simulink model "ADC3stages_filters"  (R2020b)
settings: Solver=VariableStepAuto  StartTime=0.0  StopTime=100e-3  RelTol=1e-3
libraries: ee_lib x8, fl_lib x5, nesl_utility x4, simulink_extras x2, dspmlti4 x2, simulink x1

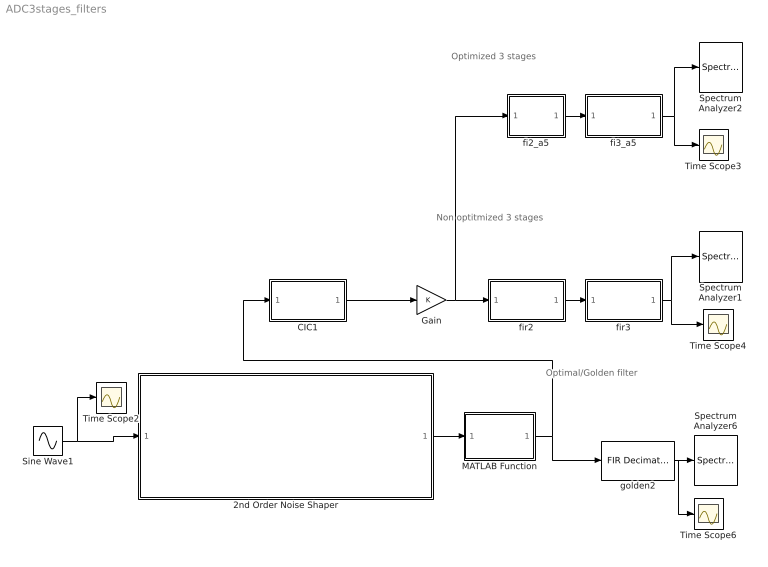
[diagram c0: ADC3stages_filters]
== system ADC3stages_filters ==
  note: Optimized 3 stages
  note: Non optitmized 3 stages
  note: Optimal/Golden filter
  2nd Order Noise Shaper : Subsystem
  CIC1 : Subsystem  Tag=BlockMethodSubSystem
  Gain : Gain  ParamDataTypeStr=int16
  MATLAB Function : MATLAB Function  TreatAsAtomicUnit=on
  Sine Wave1 : Sin  Amplitude=0.5  Bias=0.5  Frequency=2*pi*2000  SampleTime=0
  Spectrum Analyzer1 : SpectrumAnalyzer
  Spectrum Analyzer2 : SpectrumAnalyzer
  Spectrum Analyzer6 : SpectrumAnalyzer  Commented=on
  Time Scope{2..4,6} (4 alike) : Scope
  fi2_a5 : Subsystem  Tag=FilterWizardSubSystem
  fi3_a5 : Subsystem  Tag=FilterWizardSubSystem
  fir2 : Subsystem  Tag=FilterWizardSubSystem
  fir3 : Subsystem  Tag=FilterWizardSubSystem
  golden2 : dspmlti4/FIR Decimation  Tag=BlockMethodSubSystem  FilterSource=Dialog parameters  h=[-9.28934945917742932e-09 -2.06150874537475163e-09 -2.28946243433772473e-09 -2.53402570041462021e-09 -2.79572593785659298e-09 -3.07556170283654811e-09 -3.37426400279055493e-09 -3.69267761653814601e-09 -4.0317656513874688e-09 -4.39228892641005716e-09 -4.77551823656375575e-09 -5.18221175819345824e-09 -5.6139960130665323e-09 -6.07162645637982626e-09 -6.55700619397832109e-09 -7.07075410921223467e-09 -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  D=128  filtStruct=Direct form  FilterObject=FDECIM  InputProcessing=Columns as channels (frame based)  framing=Allow multirate processing  inputOffset=0  outputBufInitCond=0  roundingMode=Floor  overflowMode=off  firstCoeffDataTypeStr=Inherit: Same word length as input  firstCoeffMin=[]  firstCoeffMax=[]  firstCoeffLastDataTypeStr=Inherit: Same word length as input  outputDataTypeStr=Inherit: Same as accumulator  outputMin=[]  outputMax=[]  outputLastDataTypeStr=Inherit: Same as accumulator
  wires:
  Sine Wave1/1 -> 2nd Order Noise Shaper/1(input0), Time Scope2/1
  2nd Order Noise Shaper/1(u) -> MATLAB Function/1(u)
  golden2/1 -> Time Scope6/1, Spectrum Analyzer6/1
  MATLAB Function/1(y) -> CIC1/1(y), golden2/1
  fir2/1(Output) -> fir3/1(Input)
  fir3/1(Output) -> Spectrum Analyzer1/1, Time Scope4/1
  fi2_a5/1(Output) -> fi3_a5/1(Input)
  fi3_a5/1(Output) -> Spectrum Analyzer2/1, Time Scope3/1
  CIC1/1(Input) -> Gain/1
  Gain/1 -> fi2_a5/1(Input), fir2/1(Input)

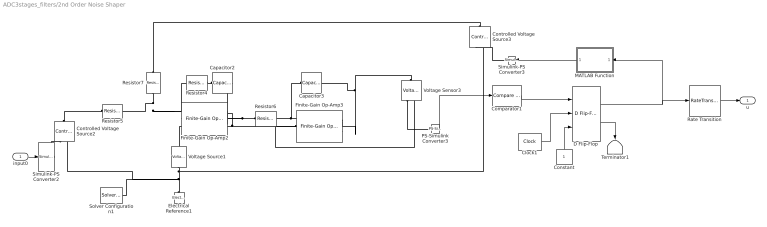
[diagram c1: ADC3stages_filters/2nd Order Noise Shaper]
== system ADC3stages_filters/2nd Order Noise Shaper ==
  input0 : Inport
  Capacitor2 : ee_lib/Passive/Capacitor  cap_option=0  c=100 pF  Cvec=[1e-05, 1e-06] F  Vvec=[0, 10] V  CV_table_symmetry=1  f_vec=[1, 10] kHz  DFext_vec=[.8, 1.2]  C_tol=5  enable_C_tol=0  tol_distribution=1  nSigma=4  r=1e-9 Ohm  g=0 1/Ohm  averaging_period=0 s  enable_operating_limits=0  operating_limit_action=2  max_working_voltage_range=[-25, 25] V  power_rating=1 W  enable_faults=0  fault_action=1  Cscale_faulted=100  R_faulted=1e-3 Ohm  G_faulted=0 1/Ohm  tau_fault=1e-3 s  enable_temporal_fault=0  t_fault=1 s  enable_behavioral_fault=0  max_permissible_voltage_range=[-100, 100] V  t_fail_on_voltage=1 s  i_specify=off  i_priority=None  i=0 A  i_nominal_specify=off  i_nominal_unit=A  i_nominal_value=1  v_specify=off  v_priority=None  v=0 V  v_nominal_specify=off  v_nominal_unit=V  v_nominal_value=1  vc_specify=off  vc_priority=High  vc=0 V  vc_nominal_specify=off  vc_nominal_unit=V  vc_nominal_value=1
  Capacitor3 : ee_lib/Passive/Capacitor  cap_option=0  c=100 pF  Cvec=[1e-05, 1e-06] F  Vvec=[0, 10] V  CV_table_symmetry=1  f_vec=[1, 10] kHz  DFext_vec=[.8, 1.2]  C_tol=5  enable_C_tol=0  tol_distribution=1  nSigma=4  r=1e-6 Ohm  g=0 1/Ohm  averaging_period=0 s  enable_operating_limits=0  operating_limit_action=2  max_working_voltage_range=[-25, 25] V  power_rating=1 W  enable_faults=0  fault_action=1  Cscale_faulted=100  R_faulted=1e-3 Ohm  G_faulted=0 1/Ohm  tau_fault=1e-3 s  enable_temporal_fault=0  t_fault=1 s  enable_behavioral_fault=0  max_permissible_voltage_range=[-100, 100] V  t_fail_on_voltage=1 s  i_specify=off  i_priority=None  i=0 A  i_nominal_specify=off  i_nominal_unit=A  i_nominal_value=1  v_specify=off  v_priority=None  v=0 V  v_nominal_specify=off  v_nominal_unit=V  v_nominal_value=1  vc_specify=off  vc_priority=High  vc=0 V  vc_nominal_specify=off  vc_nominal_unit=V  vc_nominal_value=1
  Clock1 : simulink_extras/Flip Flops/Clock  period=1/(6.25*1e6)
  Comparator1 : simulink/Logic and Bit Operations/Compare To Zero  relop=>=  OutDataTypeStr=boolean  ZeroCross=off
  Constant : Constant  SampleTime=0
  Controlled Voltage Source2 : fl_lib/Electrical/Electrical Sources/Controlled Voltage Source
  Controlled Voltage Source3 : fl_lib/Electrical/Electrical Sources/Controlled Voltage Source
  D Flip-Flop : simulink_extras/Flip Flops/D Flip-Flop
  Electrical Reference1 : fl_lib/Electrical/Electrical Elements/Electrical Reference
  Finite-Gain Op-Amp2 : ee_lib/Integrated Circuits/Finite-Gain Op-Amp  A=1000  Rin=1e6 Ohm  Rout=1 Ohm  Vmin=-1 V  Vmax=1 V  noise_mode=0  v_noise=30e-9 V/Hz^0.50000  noise_prm=1  i_noise=0.5e-12 A/Hz^0.50000  ip_noise=0.5e-12 A/Hz^0.50000  in_noise=0.5e-12 A/Hz^0.50000  sample_time=1e-3 s  repeatability=1  auto_seed_v=3499211588  auto_seed_ip=3890346746  auto_seed_in=545404223  user_seed_v=0  user_seed_ip=0  user_seed_in=0
  Finite-Gain Op-Amp3 : ee_lib/Integrated Circuits/Finite-Gain Op-Amp  A=1000  Rin=1e6 Ohm  Rout=1 Ohm  Vmin=-1 V  Vmax=1 V  noise_mode=0  v_noise=30e-9 V/Hz^0.50000  noise_prm=1  i_noise=0.5e-12 A/Hz^0.50000  ip_noise=0.5e-12 A/Hz^0.50000  in_noise=0.5e-12 A/Hz^0.50000  sample_time=1e-3 s  repeatability=1  auto_seed_v=3922919431  auto_seed_ip=2715962282  auto_seed_in=418932850  user_seed_v=0  user_seed_ip=0  user_seed_in=0
  MATLAB Function : MATLAB Function  TreatAsAtomicUnit=on
  PS-Simulink Converter3 : nesl_utility/PS-Simulink Converter  PhysicalDomain=network_engine_domain  SubClassName=ps_output  LeftPortType=input  RightPortType=output  PseudoPeriodic=off  Frequencies=[]  Unit=V  AffineConversion=off
  Rate Transition : RateTransition  OutPortSampleTime=1/(6.25e6)
  Resistor4 : fl_lib/Electrical/Electrical Elements/Resistor  R=4.304 kOhm  i_specify=off  i_priority=None  i=0 A  i_nominal_specify=off  i_nominal_unit=A  i_nominal_value=1  v_specify=off  v_priority=None  v=0 V  v_nominal_specify=off  v_nominal_unit=V  v_nominal_value=1
  Resistor5 : ee_lib/Passive/Resistor  R=4.304 kOhm  R_tol=5  enable_R_tol=0  tol_distribution=1  nSigma=4  enable_operating_limits=0  operating_limit_action=2  max_working_voltage=100 V  power_rating=1 W  enable_faults=0  fault_action=1  R_faulted=inf Ohm  enable_temporal_fault=0  t_fault=1 s  enable_behavioral_fault=0  max_permissible_current=1 A  t_fail_on_current=1 s  noise_mode=0  sample_time=1e-3 s  repeatability=1  auto_seed=1196140742  user_seed=0  Tdevice=25 degC  alpha=3.93e-3 1/K  Tmeas=25 degC  thermal_mass=100 J/K  power_derating_T1=70 degC  power_derating_T2=155 degC  operating_temperature_range_vec=[-50, 150] degC  temperature_specify=off  temperature_priority=High  temperature=298.15 K  temperature_nominal_specify=off  temperature_nominal_unit=K  temperature_nominal_value=1
  Resistor6 : ee_lib/Passive/Resistor  R=4.304 kOhm  R_tol=5  enable_R_tol=0  tol_distribution=1  nSigma=4  enable_operating_limits=0  operating_limit_action=2  max_working_voltage=100 V  power_rating=1 W  enable_faults=0  fault_action=1  R_faulted=inf Ohm  enable_temporal_fault=0  t_fault=1 s  enable_behavioral_fault=0  max_permissible_current=1 A  t_fail_on_current=1 s  noise_mode=0  sample_time=1e-3 s  repeatability=1  auto_seed=2348838240  user_seed=0  Tdevice=25 degC  alpha=3.93e-3 1/K  Tmeas=25 degC  thermal_mass=100 J/K  power_derating_T1=70 degC  power_derating_T2=155 degC  operating_temperature_range_vec=[-50, 150] degC  temperature_specify=off  temperature_priority=High  temperature=298.15 K  temperature_nominal_specify=off  temperature_nominal_unit=K  temperature_nominal_value=1
  Resistor7 : ee_lib/Passive/Resistor  R=4.304 kOhm  R_tol=5  enable_R_tol=0  tol_distribution=1  nSigma=4  enable_operating_limits=0  operating_limit_action=2  max_working_voltage=100 V  power_rating=1 W  enable_faults=0  fault_action=1  R_faulted=inf Ohm  enable_temporal_fault=0  t_fault=1 s  enable_behavioral_fault=0  max_permissible_current=1 A  t_fail_on_current=1 s  noise_mode=0  sample_time=1e-3 s  repeatability=1  auto_seed=4112460543  user_seed=0  Tdevice=25 degC  alpha=3.93e-3 1/K  Tmeas=25 degC  thermal_mass=100 J/K  power_derating_T1=70 degC  power_derating_T2=155 degC  operating_temperature_range_vec=[-50, 150] degC  temperature_specify=off  temperature_priority=High  temperature=298.15 K  temperature_nominal_specify=off  temperature_nominal_unit=K  temperature_nominal_value=1
  Simulink-PS Converter2 : nesl_utility/Simulink-PS Converter  PhysicalDomain=network_engine_domain  SubClassName=ps_input  LeftPortType=input  RightPortType=output  PseudoPeriodic=off  Frequencies=[]  NoiseDistribution=none  NoiseParameters=[]  Unit=1  AffineConversion=off  FilteringAndDerivatives=provide  SimscapeFilterOrder=1  InputFilterTimeConstant=0.001  UdotUserProvided=0
  Simulink-PS Converter3 : nesl_utility/Simulink-PS Converter  PhysicalDomain=network_engine_domain  SubClassName=ps_input  LeftPortType=input  RightPortType=output  PseudoPeriodic=off  Frequencies=[]  NoiseDistribution=none  NoiseParameters=[]  Unit=1  AffineConversion=off  FilteringAndDerivatives=provide  SimscapeFilterOrder=1  InputFilterTimeConstant=0.001  UdotUserProvided=0
  Solver Configuration1 : nesl_utility/Solver Configuration  PhysicalDomain=network_engine_domain  SubClassName=solver  LeftPortType=input  RightPortType=generic  Tones=[]  Harmonics=[]  SimulateNoise=off  Profile=off  UseLocalSampling=off  EnableSwitchedLinearOptims=on  FrequencyDomain=off  UseCCode=off  RelTol=0.001  AbsTol=1e-06  MinStep=1e-09  ToWorkspace=off  RevertToSquareIcSolve=off  NumHomotopyIterations=100  PhasorMode=off  PhasorModeNumHarmonics=1  DoDC=off  ResidualTolerance=1e-09  UseLocalSolver=off  LocalSolverChoice=NE_BACKWARD_EULER_ADVANCER  LocalSolverSampleTime=0.001  DoFixedCost=off  MaxNonlinIter=3  MaxModeIter=2  ComputeImpulses=off  ImpulseIterations=2  LinearAlgebra=auto  EquationFormulation=NE_TIME_EF  DelaysMemoryBudget=1024  AutomaticFiltering=on  FilteringTimeConstant=0.001  PartitionStorageMethod=AS_NEEDED  PartitionMemoryBudget=1024  PartitionMethod=ROBUST
  Terminator1 : Terminator
  Voltage Sensor3 : fl_lib/Electrical/Electrical Sensors/Voltage Sensor
  Voltage Source1 : ee_lib/Sources/Voltage Source  dc_voltage=0.5 V  ac_voltage=0 V  ac_shift=0 rad  ac_frequency=60 Hz  noise_mode=0  PSD=0 V^2/Hz  repeatability=1  auto_seed=4144164703  user_seed=0  sample_time=1e-3 s  i_specify=off  i_priority=None  i=0 A  i_nominal_specify=off  i_nominal_unit=A  i_nominal_value=1  v_specify=off  v_priority=None  v=0 V  v_nominal_specify=off  v_nominal_unit=V  v_nominal_value=1
  u : Outport
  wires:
  PS-Simulink Converter3/1 -> Comparator1/1
  Clock1/1 -> D Flip-Flop/2
  D Flip-Flop/1 -> MATLAB Function/1(u), Rate Transition/1
  Constant/1 -> D Flip-Flop/3
  MATLAB Function/1(y) -> Simulink-PS Converter3/1
  D Flip-Flop/2 -> Terminator1/1
  Comparator1/1 -> D Flip-Flop/1
  input0/1 -> Simulink-PS Converter2/1
  Rate Transition/1 -> u/1
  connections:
  Voltage Source1/RConn1 -- Controlled Voltage Source3/RConn2 -- Controlled Voltage Source2/RConn2 -- Solver Configuration1/RConn1 -- Electrical Reference1/LConn1
  Resistor6/LConn1 -- Capacitor2/RConn1 -- Finite-Gain Op-Amp2/RConn1
  Finite-Gain Op-Amp3/LConn1 -- Voltage Sensor3/RConn2 -- Voltage Source1/LConn1 -- Finite-Gain Op-Amp2/LConn1
  Simulink-PS Converter3/RConn1 -- Controlled Voltage Source3/RConn1
  Voltage Sensor3/LConn1 -- Capacitor3/RConn1 -- Finite-Gain Op-Amp3/RConn1
  Resistor7/RConn1 -- Resistor5/RConn1 -- Resistor4/LConn1 -- Finite-Gain Op-Amp2/LConn2
  Capacitor3/LConn1 -- Resistor6/RConn1 -- Finite-Gain Op-Amp3/LConn2
  Simulink-PS Converter2/RConn1 -- Controlled Voltage Source2/RConn1
  Voltage Sensor3/RConn1 -- PS-Simulink Converter3/LConn1
  Capacitor2/LConn1 -- Resistor4/RConn1
  Controlled Voltage Source2/LConn1 -- Resistor5/LConn1
  Controlled Voltage Source3/LConn1 -- Resistor7/LConn1

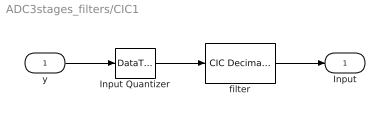
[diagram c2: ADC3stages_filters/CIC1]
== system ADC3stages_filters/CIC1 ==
  y : Inport
  Input Quantizer : DataTypeConversion  OutDataTypeStr=fixdt(1,16,15)  RndMeth=Round
  filter : dspmlti4/CIC Decimation  filtFrom=Dialog parameters  filtobj=CICDECIM  ftype=Decimator  R=32  M=1  N=2  filterInternals=Specify word lengths  BPS=[26 26 26 26]  FLPS=[15 15 15 15]  outputWordLength=14  outputFracLength=15  launchFVT=off  framing=Maintain input frame rate  RateOptions=Allow multirate processing
  Input : Outport
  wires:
  y/1 -> Input Quantizer/1
  Input Quantizer/1 -> filter/1
  filter/1 -> Input/1

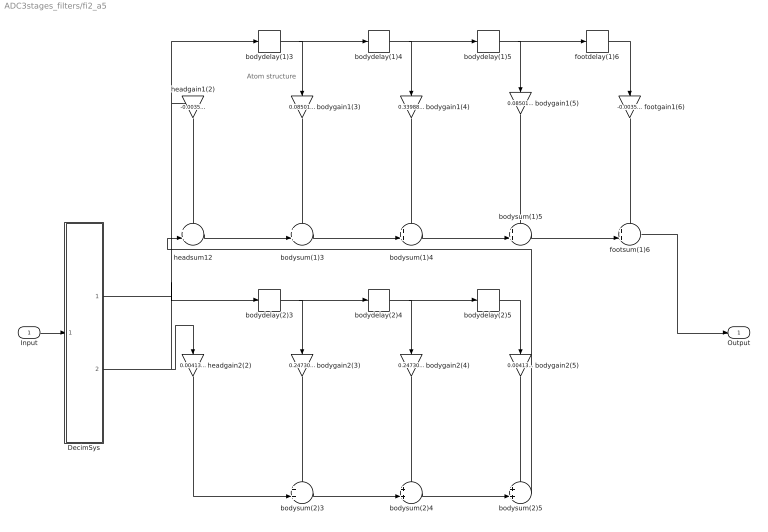
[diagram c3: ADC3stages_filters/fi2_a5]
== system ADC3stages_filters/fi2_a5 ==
  note: Atom structure
  Input : Inport
  DecimSys : Subsystem  Tag=FilterWizardDecimatorCommutator
  bodydelay(1)3 : Delay  DelayLength=1  InitialCondition=0  InputProcessing=Columns as channels (frame based)
  bodydelay(1)4 : Delay  DelayLength=1  InitialCondition=0  InputProcessing=Columns as channels (frame based)
  bodydelay(1)5 : Delay  DelayLength=1  InitialCondition=0  InputProcessing=Columns as channels (frame based)
  bodydelay(2)3 : Delay  DelayLength=1  InitialCondition=0  InputProcessing=Columns as channels (frame based)
  bodydelay(2)4 : Delay  DelayLength=1  InitialCondition=0  InputProcessing=Columns as channels (frame based)
  bodydelay(2)5 : Delay  DelayLength=1  InitialCondition=0  InputProcessing=Columns as channels (frame based)
  bodygain1(3) : Gain  Gain=0.0850178725020250964  ParamDataTypeStr=double  RndMeth=Nearest  SaturateOnIntegerOverflow=on
  bodygain1(4) : Gain  Gain=0.339887672820711306  ParamDataTypeStr=double  RndMeth=Nearest  SaturateOnIntegerOverflow=on
  bodygain1(5) : Gain  Gain=0.0850178725020250964  ParamDataTypeStr=double  RndMeth=Nearest  SaturateOnIntegerOverflow=on
  bodygain2(3) : Gain  Gain=0.247309117408189227  ParamDataTypeStr=double  RndMeth=Nearest  SaturateOnIntegerOverflow=on
  bodygain2(4) : Gain  Gain=0.247309117408189227  ParamDataTypeStr=double  RndMeth=Nearest  SaturateOnIntegerOverflow=on
  bodygain2(5) : Gain  Gain=0.00413248237921627366  ParamDataTypeStr=double  RndMeth=Nearest  SaturateOnIntegerOverflow=on
  bodysum(1)3 : Sum  Inputs=++|  RndMeth=Nearest  SaturateOnIntegerOverflow=on
  bodysum(1)4 : Sum  Inputs=++|  RndMeth=Nearest  SaturateOnIntegerOverflow=on
  bodysum(1)5 : Sum  Inputs=++|  RndMeth=Nearest  SaturateOnIntegerOverflow=on
  bodysum(2)3 : Sum  Inputs=++|  RndMeth=Nearest  SaturateOnIntegerOverflow=on
  bodysum(2)4 : Sum  Inputs=++|  RndMeth=Nearest  SaturateOnIntegerOverflow=on
  bodysum(2)5 : Sum  Inputs=++|  RndMeth=Nearest  SaturateOnIntegerOverflow=on
  footdelay(1)6 : Delay  DelayLength=1  InitialCondition=0  InputProcessing=Columns as channels (frame based)
  footgain1(6) : Gain  Gain=-0.00352510912497529033  ParamDataTypeStr=double  RndMeth=Nearest  SaturateOnIntegerOverflow=on
  footsum(1)6 : Sum  Inputs=++|  RndMeth=Nearest  SaturateOnIntegerOverflow=on
  headgain1(2) : Gain  Gain=-0.00352510912497529033  ParamDataTypeStr=double  RndMeth=Nearest  SaturateOnIntegerOverflow=on
  headgain2(2) : Gain  Gain=0.00413248237921627366  ParamDataTypeStr=double  RndMeth=Nearest  SaturateOnIntegerOverflow=on
  headsum12 : Sum  Inputs=++|  RndMeth=Nearest  SaturateOnIntegerOverflow=on
  Output : Outport
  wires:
  Input/1 -> DecimSys/1(input)
  DecimSys/1(output1) -> headgain1(2)/1, bodydelay(1)3/1
  DecimSys/2(output2) -> headgain2(2)/1, bodydelay(2)3/1
  headgain1(2)/1 -> headsum12/1
  headgain2(2)/1 -> bodysum(2)3/2
  headsum12/1 -> bodysum(1)3/2
  bodygain1(3)/1 -> bodysum(1)3/1
  bodygain2(3)/1 -> bodysum(2)3/1
  bodysum(1)3/1 -> bodysum(1)4/2
  bodysum(2)3/1 -> bodysum(2)4/2
  bodydelay(1)3/1 -> bodygain1(3)/1, bodydelay(1)4/1
  bodydelay(2)3/1 -> bodygain2(3)/1, bodydelay(2)4/1
  bodygain1(4)/1 -> bodysum(1)4/1
  bodygain2(4)/1 -> bodysum(2)4/1
  bodysum(1)4/1 -> bodysum(1)5/2
  bodysum(2)4/1 -> bodysum(2)5/2
  bodydelay(1)4/1 -> bodygain1(4)/1, bodydelay(1)5/1
  bodydelay(2)4/1 -> bodygain2(4)/1, bodydelay(2)5/1
  bodygain1(5)/1 -> bodysum(1)5/1
  bodygain2(5)/1 -> bodysum(2)5/1
  bodysum(1)5/1 -> footsum(1)6/2
  bodysum(2)5/1 -> headsum12/2
  bodydelay(1)5/1 -> bodygain1(5)/1, footdelay(1)6/1
  bodydelay(2)5/1 -> bodygain2(5)/1
  footgain1(6)/1 -> footsum(1)6/1
  footsum(1)6/1 -> Output/1
  footdelay(1)6/1 -> footgain1(6)/1

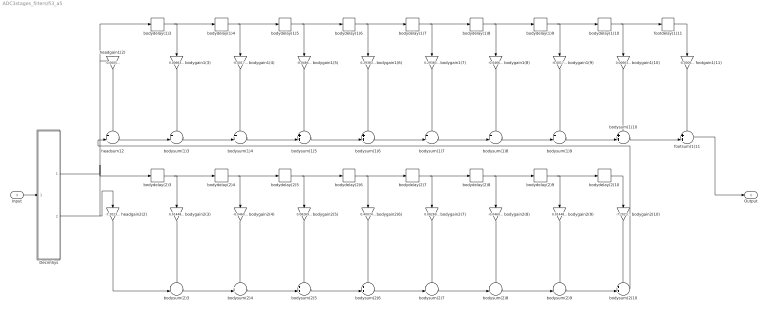
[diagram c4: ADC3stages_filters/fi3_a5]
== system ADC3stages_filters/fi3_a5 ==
  Input : Inport
  DecimSys : Subsystem  Tag=FilterWizardDecimatorCommutator
  bodydelay(1){3..10} (8 alike) : Delay  DelayLength=1  InitialCondition=0  InputProcessing=Columns as channels (frame based)
  bodydelay(2){3..10} (8 alike) : Delay  DelayLength=1  InitialCondition=0  InputProcessing=Columns as channels (frame based)
  bodygain1(10) : Gain  Gain=0.00663105967506261249  ParamDataTypeStr=double  RndMeth=Nearest  SaturateOnIntegerOverflow=on
  bodygain1(3) : Gain  Gain=0.00663105967506261249  ParamDataTypeStr=double  RndMeth=Nearest  SaturateOnIntegerOverflow=on
  bodygain1(4) : Gain  Gain=-0.0017964116772036067  ParamDataTypeStr=double  RndMeth=Nearest  SaturateOnIntegerOverflow=on
  bodygain1(5) : Gain  Gain=-0.0466786883554543702  ParamDataTypeStr=double  RndMeth=Nearest  SaturateOnIntegerOverflow=on
  bodygain1(6) : Gain  Gain=0.293833196601604174  ParamDataTypeStr=double  RndMeth=Nearest  SaturateOnIntegerOverflow=on
  bodygain1(7) : Gain  Gain=0.293833196601604174  ParamDataTypeStr=double  RndMeth=Nearest  SaturateOnIntegerOverflow=on
  bodygain1(8) : Gain  Gain=-0.0466786883554543702  ParamDataTypeStr=double  RndMeth=Nearest  SaturateOnIntegerOverflow=on
  bodygain1(9) : Gain  Gain=-0.0017964116772036067  ParamDataTypeStr=double  RndMeth=Nearest  SaturateOnIntegerOverflow=on
  bodygain2(10) : Gain  Gain=-7.20232768288544341e-05  ParamDataTypeStr=double  RndMeth=Nearest  SaturateOnIntegerOverflow=on
  bodygain2(3) : Gain  Gain=0.0144802685760407664  ParamDataTypeStr=double  RndMeth=Nearest  SaturateOnIntegerOverflow=on
  bodygain2(4) : Gain  Gain=-0.0460334870391839596  ParamDataTypeStr=double  RndMeth=Nearest  SaturateOnIntegerOverflow=on
  bodygain2(5) : Gain  Gain=0.0826995303354833844  ParamDataTypeStr=double  RndMeth=Nearest  SaturateOnIntegerOverflow=on
  bodygain2(6) : Gain  Gain=0.400745433772089155  ParamDataTypeStr=double  RndMeth=Nearest  SaturateOnIntegerOverflow=on
  bodygain2(7) : Gain  Gain=0.0826995303354833844  ParamDataTypeStr=double  RndMeth=Nearest  SaturateOnIntegerOverflow=on
  bodygain2(8) : Gain  Gain=-0.0460334870391839596  ParamDataTypeStr=double  RndMeth=Nearest  SaturateOnIntegerOverflow=on
  bodygain2(9) : Gain  Gain=0.0144802685760407664  ParamDataTypeStr=double  RndMeth=Nearest  SaturateOnIntegerOverflow=on
  bodysum(1){3..10} (8 alike) : Sum  Inputs=++|  RndMeth=Nearest  SaturateOnIntegerOverflow=on
  bodysum(2){3..10} (8 alike) : Sum  Inputs=++|  RndMeth=Nearest  SaturateOnIntegerOverflow=on
  footdelay(1)11 : Delay  DelayLength=1  InitialCondition=0  InputProcessing=Columns as channels (frame based)
  footgain1(11) : Gain  Gain=-0.000557962150753790048  ParamDataTypeStr=double  RndMeth=Nearest  SaturateOnIntegerOverflow=on
  footsum(1)11 : Sum  Inputs=++|  RndMeth=Nearest  SaturateOnIntegerOverflow=on
  headgain1(2) : Gain  Gain=-0.000557962150753790048  ParamDataTypeStr=double  RndMeth=Nearest  SaturateOnIntegerOverflow=on
  headgain2(2) : Gain  Gain=-7.20232768288544341e-05  ParamDataTypeStr=double  RndMeth=Nearest  SaturateOnIntegerOverflow=on
  headsum12 : Sum  Inputs=++|  RndMeth=Nearest  SaturateOnIntegerOverflow=on
  Output : Outport
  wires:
  Input/1 -> DecimSys/1(input)
  DecimSys/1(output1) -> headgain1(2)/1, bodydelay(1)3/1
  DecimSys/2(output2) -> headgain2(2)/1, bodydelay(2)3/1
  headgain1(2)/1 -> headsum12/1
  headgain2(2)/1 -> bodysum(2)3/2
  headsum12/1 -> bodysum(1)3/2
  bodygain1(3)/1 -> bodysum(1)3/1
  bodygain2(3)/1 -> bodysum(2)3/1
  bodysum(1)3/1 -> bodysum(1)4/2
  bodysum(2)3/1 -> bodysum(2)4/2
  bodydelay(1)3/1 -> bodygain1(3)/1, bodydelay(1)4/1
  bodydelay(2)3/1 -> bodygain2(3)/1, bodydelay(2)4/1
  bodygain1(4)/1 -> bodysum(1)4/1
  bodygain2(4)/1 -> bodysum(2)4/1
  bodysum(1)4/1 -> bodysum(1)5/2
  bodysum(2)4/1 -> bodysum(2)5/2
  bodydelay(1)4/1 -> bodygain1(4)/1, bodydelay(1)5/1
  bodydelay(2)4/1 -> bodygain2(4)/1, bodydelay(2)5/1
  bodygain1(5)/1 -> bodysum(1)5/1
  bodygain2(5)/1 -> bodysum(2)5/1
  bodysum(1)5/1 -> bodysum(1)6/2
  bodysum(2)5/1 -> bodysum(2)6/2
  bodydelay(1)5/1 -> bodygain1(5)/1, bodydelay(1)6/1
  bodydelay(2)5/1 -> bodygain2(5)/1, bodydelay(2)6/1
  bodygain1(6)/1 -> bodysum(1)6/1
  bodygain2(6)/1 -> bodysum(2)6/1
  bodysum(1)6/1 -> bodysum(1)7/2
  bodysum(2)6/1 -> bodysum(2)7/2
  bodydelay(1)6/1 -> bodygain1(6)/1, bodydelay(1)7/1
  bodydelay(2)6/1 -> bodygain2(6)/1, bodydelay(2)7/1
  bodygain1(7)/1 -> bodysum(1)7/1
  bodygain2(7)/1 -> bodysum(2)7/1
  bodysum(1)7/1 -> bodysum(1)8/2
  bodysum(2)7/1 -> bodysum(2)8/2
  bodydelay(1)7/1 -> bodygain1(7)/1, bodydelay(1)8/1
  bodydelay(2)7/1 -> bodygain2(7)/1, bodydelay(2)8/1
  bodygain1(8)/1 -> bodysum(1)8/1
  bodygain2(8)/1 -> bodysum(2)8/1
  bodysum(1)8/1 -> bodysum(1)9/2
  bodysum(2)8/1 -> bodysum(2)9/2
  bodydelay(1)8/1 -> bodygain1(8)/1, bodydelay(1)9/1
  bodydelay(2)8/1 -> bodygain2(8)/1, bodydelay(2)9/1
  bodygain1(9)/1 -> bodysum(1)9/1
  bodygain2(9)/1 -> bodysum(2)9/1
  bodysum(1)9/1 -> bodysum(1)10/2
  bodysum(2)9/1 -> bodysum(2)10/2
  bodydelay(1)9/1 -> bodygain1(9)/1, bodydelay(1)10/1
  bodydelay(2)9/1 -> bodygain2(9)/1, bodydelay(2)10/1
  bodygain1(10)/1 -> bodysum(1)10/1
  bodygain2(10)/1 -> bodysum(2)10/1
  bodysum(1)10/1 -> footsum(1)11/2
  bodysum(2)10/1 -> headsum12/2
  bodydelay(1)10/1 -> bodygain1(10)/1, footdelay(1)11/1
  bodydelay(2)10/1 -> bodygain2(10)/1
  footgain1(11)/1 -> footsum(1)11/1
  footsum(1)11/1 -> Output/1
  footdelay(1)11/1 -> footgain1(11)/1

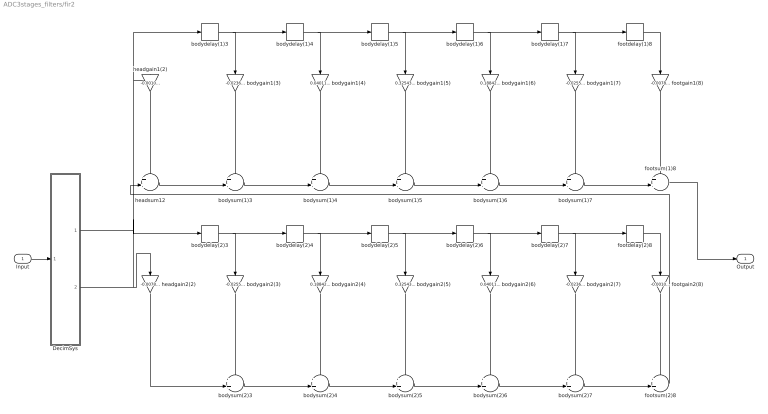
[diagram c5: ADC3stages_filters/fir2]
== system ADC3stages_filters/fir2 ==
  Input : Inport
  DecimSys : Subsystem  Tag=FilterWizardDecimatorCommutator
  bodydelay(1){3..7} (5 alike) : Delay  DelayLength=1  InitialCondition=0  InputProcessing=Columns as channels (frame based)
  bodydelay(2){3..7} (5 alike) : Delay  DelayLength=1  InitialCondition=0  InputProcessing=Columns as channels (frame based)
  bodygain1(3) : Gain  Gain=-0.0236575305385687412  ParamDataTypeStr=double  RndMeth=Nearest  SaturateOnIntegerOverflow=on
  bodygain1(4) : Gain  Gain=0.0401106064947036045  ParamDataTypeStr=double  RndMeth=Nearest  SaturateOnIntegerOverflow=on
  bodygain1(5) : Gain  Gain=0.325434987422980881  ParamDataTypeStr=double  RndMeth=Nearest  SaturateOnIntegerOverflow=on
  bodygain1(6) : Gain  Gain=0.188427753939350962  ParamDataTypeStr=double  RndMeth=Nearest  SaturateOnIntegerOverflow=on
  bodygain1(7) : Gain  Gain=-0.0255620476687289794  ParamDataTypeStr=double  RndMeth=Nearest  SaturateOnIntegerOverflow=on
  bodygain2(3) : Gain  Gain=-0.0255620476687289794  ParamDataTypeStr=double  RndMeth=Nearest  SaturateOnIntegerOverflow=on
  bodygain2(4) : Gain  Gain=0.188427753939350962  ParamDataTypeStr=double  RndMeth=Nearest  SaturateOnIntegerOverflow=on
  bodygain2(5) : Gain  Gain=0.325434987422980881  ParamDataTypeStr=double  RndMeth=Nearest  SaturateOnIntegerOverflow=on
  bodygain2(6) : Gain  Gain=0.0401106064947036045  ParamDataTypeStr=double  RndMeth=Nearest  SaturateOnIntegerOverflow=on
  bodygain2(7) : Gain  Gain=-0.0236575305385687412  ParamDataTypeStr=double  RndMeth=Nearest  SaturateOnIntegerOverflow=on
  bodysum(1){3..7} (5 alike) : Sum  Inputs=++|  RndMeth=Nearest  SaturateOnIntegerOverflow=on
  bodysum(2){3..7} (5 alike) : Sum  Inputs=++|  RndMeth=Nearest  SaturateOnIntegerOverflow=on
  footdelay(1)8 : Delay  DelayLength=1  InitialCondition=0  InputProcessing=Columns as channels (frame based)
  footdelay(2)8 : Delay  DelayLength=1  InitialCondition=0  InputProcessing=Columns as channels (frame based)
  footgain1(8) : Gain  Gain=-0.0078736214127589528  ParamDataTypeStr=double  RndMeth=Nearest  SaturateOnIntegerOverflow=on
  footgain2(8) : Gain  Gain=-0.00102546363558656635  ParamDataTypeStr=double  RndMeth=Nearest  SaturateOnIntegerOverflow=on
  footsum(1)8 : Sum  Inputs=++|  RndMeth=Nearest  SaturateOnIntegerOverflow=on
  footsum(2)8 : Sum  Inputs=++|  RndMeth=Nearest  SaturateOnIntegerOverflow=on
  headgain1(2) : Gain  Gain=-0.00102546363558656635  ParamDataTypeStr=double  RndMeth=Nearest  SaturateOnIntegerOverflow=on
  headgain2(2) : Gain  Gain=-0.0078736214127589528  ParamDataTypeStr=double  RndMeth=Nearest  SaturateOnIntegerOverflow=on
  headsum12 : Sum  Inputs=++|  RndMeth=Nearest  SaturateOnIntegerOverflow=on
  Output : Outport
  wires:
  Input/1 -> DecimSys/1(input)
  DecimSys/1(output1) -> headgain1(2)/1, bodydelay(1)3/1
  DecimSys/2(output2) -> headgain2(2)/1, bodydelay(2)3/1
  headgain1(2)/1 -> headsum12/1
  headgain2(2)/1 -> bodysum(2)3/2
  headsum12/1 -> bodysum(1)3/2
  bodygain1(3)/1 -> bodysum(1)3/1
  bodygain2(3)/1 -> bodysum(2)3/1
  bodysum(1)3/1 -> bodysum(1)4/2
  bodysum(2)3/1 -> bodysum(2)4/2
  bodydelay(1)3/1 -> bodygain1(3)/1, bodydelay(1)4/1
  bodydelay(2)3/1 -> bodygain2(3)/1, bodydelay(2)4/1
  bodygain1(4)/1 -> bodysum(1)4/1
  bodygain2(4)/1 -> bodysum(2)4/1
  bodysum(1)4/1 -> bodysum(1)5/2
  bodysum(2)4/1 -> bodysum(2)5/2
  bodydelay(1)4/1 -> bodygain1(4)/1, bodydelay(1)5/1
  bodydelay(2)4/1 -> bodygain2(4)/1, bodydelay(2)5/1
  bodygain1(5)/1 -> bodysum(1)5/1
  bodygain2(5)/1 -> bodysum(2)5/1
  bodysum(1)5/1 -> bodysum(1)6/2
  bodysum(2)5/1 -> bodysum(2)6/2
  bodydelay(1)5/1 -> bodygain1(5)/1, bodydelay(1)6/1
  bodydelay(2)5/1 -> bodygain2(5)/1, bodydelay(2)6/1
  bodygain1(6)/1 -> bodysum(1)6/1
  bodygain2(6)/1 -> bodysum(2)6/1
  bodysum(1)6/1 -> bodysum(1)7/2
  bodysum(2)6/1 -> bodysum(2)7/2
  bodydelay(1)6/1 -> bodygain1(6)/1, bodydelay(1)7/1
  bodydelay(2)6/1 -> bodygain2(6)/1, bodydelay(2)7/1
  bodygain1(7)/1 -> bodysum(1)7/1
  bodygain2(7)/1 -> bodysum(2)7/1
  bodysum(1)7/1 -> footsum(1)8/2
  bodysum(2)7/1 -> footsum(2)8/2
  bodydelay(1)7/1 -> bodygain1(7)/1, footdelay(1)8/1
  bodydelay(2)7/1 -> bodygain2(7)/1, footdelay(2)8/1
  footgain1(8)/1 -> footsum(1)8/1
  footgain2(8)/1 -> footsum(2)8/1
  footsum(1)8/1 -> Output/1
  footsum(2)8/1 -> headsum12/2
  footdelay(1)8/1 -> footgain1(8)/1
  footdelay(2)8/1 -> footgain2(8)/1

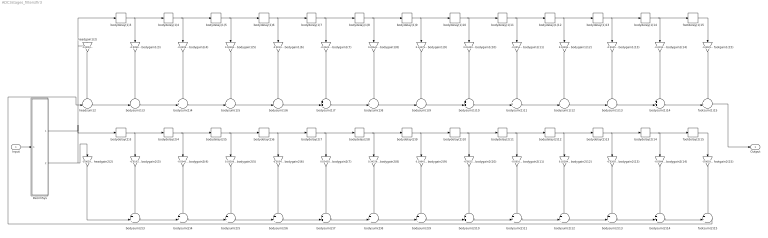
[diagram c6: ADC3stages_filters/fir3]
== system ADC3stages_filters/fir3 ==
  Input : Inport
  DecimSys : Subsystem  Tag=FilterWizardDecimatorCommutator
  bodydelay(1){3..14} (12 alike) : Delay  DelayLength=1  InitialCondition=0  InputProcessing=Columns as channels (frame based)
  bodydelay(2){3..14} (12 alike) : Delay  DelayLength=1  InitialCondition=0  InputProcessing=Columns as channels (frame based)
  bodygain1(10) : Gain  Gain=0.0342076800982699242  ParamDataTypeStr=double  RndMeth=Nearest  SaturateOnIntegerOverflow=on
  bodygain1(11) : Gain  Gain=-0.0554502205627716432  ParamDataTypeStr=double  RndMeth=Nearest  SaturateOnIntegerOverflow=on
  bodygain1(12) : Gain  Gain=0.0320648096871725546  ParamDataTypeStr=double  RndMeth=Nearest  SaturateOnIntegerOverflow=on
  bodygain1(13) : Gain  Gain=-0.00454438945123436001  ParamDataTypeStr=double  RndMeth=Nearest  SaturateOnIntegerOverflow=on
  bodygain1(14) : Gain  Gain=-0.0193627699547582119  ParamDataTypeStr=double  RndMeth=Nearest  SaturateOnIntegerOverflow=on
  bodygain1(3) : Gain  Gain=-0.00999151794139211021  ParamDataTypeStr=double  RndMeth=Nearest  SaturateOnIntegerOverflow=on
  bodygain1(4) : Gain  Gain=-0.0209497691909231072  ParamDataTypeStr=double  RndMeth=Nearest  SaturateOnIntegerOverflow=on
  bodygain1(5) : Gain  Gain=0.0228433374247001553  ParamDataTypeStr=double  RndMeth=Nearest  SaturateOnIntegerOverflow=on
  bodygain1(6) : Gain  Gain=-0.00108810484526418623  ParamDataTypeStr=double  RndMeth=Nearest  SaturateOnIntegerOverflow=on
  bodygain1(7) : Gain  Gain=-0.0623644231842223479  ParamDataTypeStr=double  RndMeth=Nearest  SaturateOnIntegerOverflow=on
  bodygain1(8) : Gain  Gain=0.206411746382430594  ParamDataTypeStr=double  RndMeth=Nearest  SaturateOnIntegerOverflow=on
  bodygain1(9) : Gain  Gain=0.343793609883162155  ParamDataTypeStr=double  RndMeth=Nearest  SaturateOnIntegerOverflow=on
  bodygain2(10) : Gain  Gain=-0.0623644231842223479  ParamDataTypeStr=double  RndMeth=Nearest  SaturateOnIntegerOverflow=on
  bodygain2(11) : Gain  Gain=-0.00108810484526418623  ParamDataTypeStr=double  RndMeth=Nearest  SaturateOnIntegerOverflow=on
  bodygain2(12) : Gain  Gain=0.0228433374247001553  ParamDataTypeStr=double  RndMeth=Nearest  SaturateOnIntegerOverflow=on
  bodygain2(13) : Gain  Gain=-0.0209497691909231072  ParamDataTypeStr=double  RndMeth=Nearest  SaturateOnIntegerOverflow=on
  bodygain2(14) : Gain  Gain=-0.00999151794139211021  ParamDataTypeStr=double  RndMeth=Nearest  SaturateOnIntegerOverflow=on
  bodygain2(3) : Gain  Gain=-0.0193627699547582119  ParamDataTypeStr=double  RndMeth=Nearest  SaturateOnIntegerOverflow=on
  bodygain2(4) : Gain  Gain=-0.00454438945123436001  ParamDataTypeStr=double  RndMeth=Nearest  SaturateOnIntegerOverflow=on
  bodygain2(5) : Gain  Gain=0.0320648096871725546  ParamDataTypeStr=double  RndMeth=Nearest  SaturateOnIntegerOverflow=on
  bodygain2(6) : Gain  Gain=-0.0554502205627716432  ParamDataTypeStr=double  RndMeth=Nearest  SaturateOnIntegerOverflow=on
  bodygain2(7) : Gain  Gain=0.0342076800982699242  ParamDataTypeStr=double  RndMeth=Nearest  SaturateOnIntegerOverflow=on
  bodygain2(8) : Gain  Gain=0.343793609883162155  ParamDataTypeStr=double  RndMeth=Nearest  SaturateOnIntegerOverflow=on
  bodygain2(9) : Gain  Gain=0.206411746382430594  ParamDataTypeStr=double  RndMeth=Nearest  SaturateOnIntegerOverflow=on
  bodysum(1){3..14} (12 alike) : Sum  Inputs=++|  RndMeth=Nearest  SaturateOnIntegerOverflow=on
  bodysum(2){3..14} (12 alike) : Sum  Inputs=++|  RndMeth=Nearest  SaturateOnIntegerOverflow=on
  footdelay(1)15 : Delay  DelayLength=1  InitialCondition=0  InputProcessing=Columns as channels (frame based)
  footdelay(2)15 : Delay  DelayLength=1  InitialCondition=0  InputProcessing=Columns as channels (frame based)
  footgain1(15) : Gain  Gain=-0.00292874486601404829  ParamDataTypeStr=double  RndMeth=Nearest  SaturateOnIntegerOverflow=on
  footgain2(15) : Gain  Gain=-0.00034773072834701522  ParamDataTypeStr=double  RndMeth=Nearest  SaturateOnIntegerOverflow=on
  footsum(1)15 : Sum  Inputs=++|  RndMeth=Nearest  SaturateOnIntegerOverflow=on
  footsum(2)15 : Sum  Inputs=++|  RndMeth=Nearest  SaturateOnIntegerOverflow=on
  headgain1(2) : Gain  Gain=-0.00034773072834701522  ParamDataTypeStr=double  RndMeth=Nearest  SaturateOnIntegerOverflow=on
  headgain2(2) : Gain  Gain=-0.00292874486601404829  ParamDataTypeStr=double  RndMeth=Nearest  SaturateOnIntegerOverflow=on
  headsum12 : Sum  Inputs=++|  RndMeth=Nearest  SaturateOnIntegerOverflow=on
  Output : Outport
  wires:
  Input/1 -> DecimSys/1(input)
  DecimSys/1(output1) -> headgain1(2)/1, bodydelay(1)3/1
  DecimSys/2(output2) -> headgain2(2)/1, bodydelay(2)3/1
  headgain1(2)/1 -> headsum12/1
  headgain2(2)/1 -> bodysum(2)3/2
  headsum12/1 -> bodysum(1)3/2
  bodygain1(3)/1 -> bodysum(1)3/1
  bodygain2(3)/1 -> bodysum(2)3/1
  bodysum(1)3/1 -> bodysum(1)4/2
  bodysum(2)3/1 -> bodysum(2)4/2
  bodydelay(1)3/1 -> bodygain1(3)/1, bodydelay(1)4/1
  bodydelay(2)3/1 -> bodygain2(3)/1, bodydelay(2)4/1
  bodygain1(4)/1 -> bodysum(1)4/1
  bodygain2(4)/1 -> bodysum(2)4/1
  bodysum(1)4/1 -> bodysum(1)5/2
  bodysum(2)4/1 -> bodysum(2)5/2
  bodydelay(1)4/1 -> bodygain1(4)/1, bodydelay(1)5/1
  bodydelay(2)4/1 -> bodygain2(4)/1, bodydelay(2)5/1
  bodygain1(5)/1 -> bodysum(1)5/1
  bodygain2(5)/1 -> bodysum(2)5/1
  bodysum(1)5/1 -> bodysum(1)6/2
  bodysum(2)5/1 -> bodysum(2)6/2
  bodydelay(1)5/1 -> bodygain1(5)/1, bodydelay(1)6/1
  bodydelay(2)5/1 -> bodygain2(5)/1, bodydelay(2)6/1
  bodygain1(6)/1 -> bodysum(1)6/1
  bodygain2(6)/1 -> bodysum(2)6/1
  bodysum(1)6/1 -> bodysum(1)7/2
  bodysum(2)6/1 -> bodysum(2)7/2
  bodydelay(1)6/1 -> bodygain1(6)/1, bodydelay(1)7/1
  bodydelay(2)6/1 -> bodygain2(6)/1, bodydelay(2)7/1
  bodygain1(7)/1 -> bodysum(1)7/1
  bodygain2(7)/1 -> bodysum(2)7/1
  bodysum(1)7/1 -> bodysum(1)8/2
  bodysum(2)7/1 -> bodysum(2)8/2
  bodydelay(1)7/1 -> bodygain1(7)/1, bodydelay(1)8/1
  bodydelay(2)7/1 -> bodygain2(7)/1, bodydelay(2)8/1
  bodygain1(8)/1 -> bodysum(1)8/1
  bodygain2(8)/1 -> bodysum(2)8/1
  bodysum(1)8/1 -> bodysum(1)9/2
  bodysum(2)8/1 -> bodysum(2)9/2
  bodydelay(1)8/1 -> bodygain1(8)/1, bodydelay(1)9/1
  bodydelay(2)8/1 -> bodygain2(8)/1, bodydelay(2)9/1
  bodygain1(9)/1 -> bodysum(1)9/1
  bodygain2(9)/1 -> bodysum(2)9/1
  bodysum(1)9/1 -> bodysum(1)10/2
  bodysum(2)9/1 -> bodysum(2)10/2
  bodydelay(1)9/1 -> bodygain1(9)/1, bodydelay(1)10/1
  bodydelay(2)9/1 -> bodygain2(9)/1, bodydelay(2)10/1
  bodygain1(10)/1 -> bodysum(1)10/1
  bodygain2(10)/1 -> bodysum(2)10/1
  bodysum(1)10/1 -> bodysum(1)11/2
  bodysum(2)10/1 -> bodysum(2)11/2
  bodydelay(1)10/1 -> bodygain1(10)/1, bodydelay(1)11/1
  bodydelay(2)10/1 -> bodygain2(10)/1, bodydelay(2)11/1
  bodygain1(11)/1 -> bodysum(1)11/1
  bodygain2(11)/1 -> bodysum(2)11/1
  bodysum(1)11/1 -> bodysum(1)12/2
  bodysum(2)11/1 -> bodysum(2)12/2
  bodydelay(1)11/1 -> bodygain1(11)/1, bodydelay(1)12/1
  bodydelay(2)11/1 -> bodygain2(11)/1, bodydelay(2)12/1
  bodygain1(12)/1 -> bodysum(1)12/1
  bodygain2(12)/1 -> bodysum(2)12/1
  bodysum(1)12/1 -> bodysum(1)13/2
  bodysum(2)12/1 -> bodysum(2)13/2
  bodydelay(1)12/1 -> bodygain1(12)/1, bodydelay(1)13/1
  bodydelay(2)12/1 -> bodygain2(12)/1, bodydelay(2)13/1
  bodygain1(13)/1 -> bodysum(1)13/1
  bodygain2(13)/1 -> bodysum(2)13/1
  bodysum(1)13/1 -> bodysum(1)14/2
  bodysum(2)13/1 -> bodysum(2)14/2
  bodydelay(1)13/1 -> bodygain1(13)/1, bodydelay(1)14/1
  bodydelay(2)13/1 -> bodygain2(13)/1, bodydelay(2)14/1
  bodygain1(14)/1 -> bodysum(1)14/1
  bodygain2(14)/1 -> bodysum(2)14/1
  bodysum(1)14/1 -> footsum(1)15/2
  bodysum(2)14/1 -> footsum(2)15/2
  bodydelay(1)14/1 -> bodygain1(14)/1, footdelay(1)15/1
  bodydelay(2)14/1 -> bodygain2(14)/1, footdelay(2)15/1
  footgain1(15)/1 -> footsum(1)15/1
  footgain2(15)/1 -> footsum(2)15/1
  footsum(1)15/1 -> Output/1
  footsum(2)15/1 -> headsum12/2
  footdelay(1)15/1 -> footgain1(15)/1
  footdelay(2)15/1 -> footgain2(15)/1

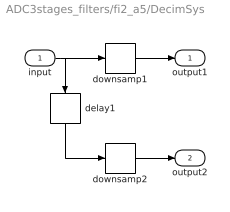
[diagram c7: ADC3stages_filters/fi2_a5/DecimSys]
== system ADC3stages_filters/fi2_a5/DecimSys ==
  input : Inport
  delay1 : Delay  DelayLength=1  InputProcessing=Columns as channels (frame based)
  downsamp1 : DownSample  RateOptions=Allow multirate processing
  downsamp2 : DownSample  RateOptions=Allow multirate processing
  output1 : Outport
  output2 : Outport  Port=2
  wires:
  input/1 -> downsamp1/1, delay1/1
  downsamp1/1 -> output1/1
  delay1/1 -> downsamp2/1
  downsamp2/1 -> output2/1

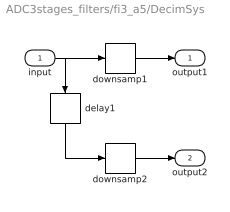
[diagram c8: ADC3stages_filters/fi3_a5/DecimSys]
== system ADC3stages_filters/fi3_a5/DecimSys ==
  input : Inport
  delay1 : Delay  DelayLength=1  InputProcessing=Columns as channels (frame based)
  downsamp1 : DownSample  RateOptions=Allow multirate processing
  downsamp2 : DownSample  RateOptions=Allow multirate processing
  output1 : Outport
  output2 : Outport  Port=2
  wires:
  input/1 -> downsamp1/1, delay1/1
  downsamp1/1 -> output1/1
  delay1/1 -> downsamp2/1
  downsamp2/1 -> output2/1

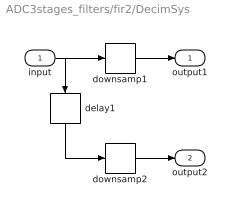
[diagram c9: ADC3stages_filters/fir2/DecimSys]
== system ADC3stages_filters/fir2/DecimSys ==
  input : Inport
  delay1 : Delay  DelayLength=1  InputProcessing=Columns as channels (frame based)
  downsamp1 : DownSample  RateOptions=Allow multirate processing
  downsamp2 : DownSample  RateOptions=Allow multirate processing
  output1 : Outport
  output2 : Outport  Port=2
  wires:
  input/1 -> downsamp1/1, delay1/1
  downsamp1/1 -> output1/1
  delay1/1 -> downsamp2/1
  downsamp2/1 -> output2/1

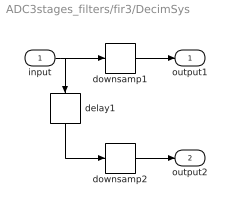
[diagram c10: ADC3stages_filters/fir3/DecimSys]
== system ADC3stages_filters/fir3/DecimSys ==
  input : Inport
  delay1 : Delay  DelayLength=1  InputProcessing=Columns as channels (frame based)
  downsamp1 : DownSample  RateOptions=Allow multirate processing
  downsamp2 : DownSample  RateOptions=Allow multirate processing
  output1 : Outport
  output2 : Outport  Port=2
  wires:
  input/1 -> downsamp1/1, delay1/1
  downsamp1/1 -> output1/1
  delay1/1 -> downsamp2/1
  downsamp2/1 -> output2/1

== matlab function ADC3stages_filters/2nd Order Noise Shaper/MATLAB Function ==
function y = inverter(u)
if u
    y = 0;
else
    y = 1;
end

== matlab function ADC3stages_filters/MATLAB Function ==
function y = bool2int(u)
if u
    y=1;
else
    y=0;
end
